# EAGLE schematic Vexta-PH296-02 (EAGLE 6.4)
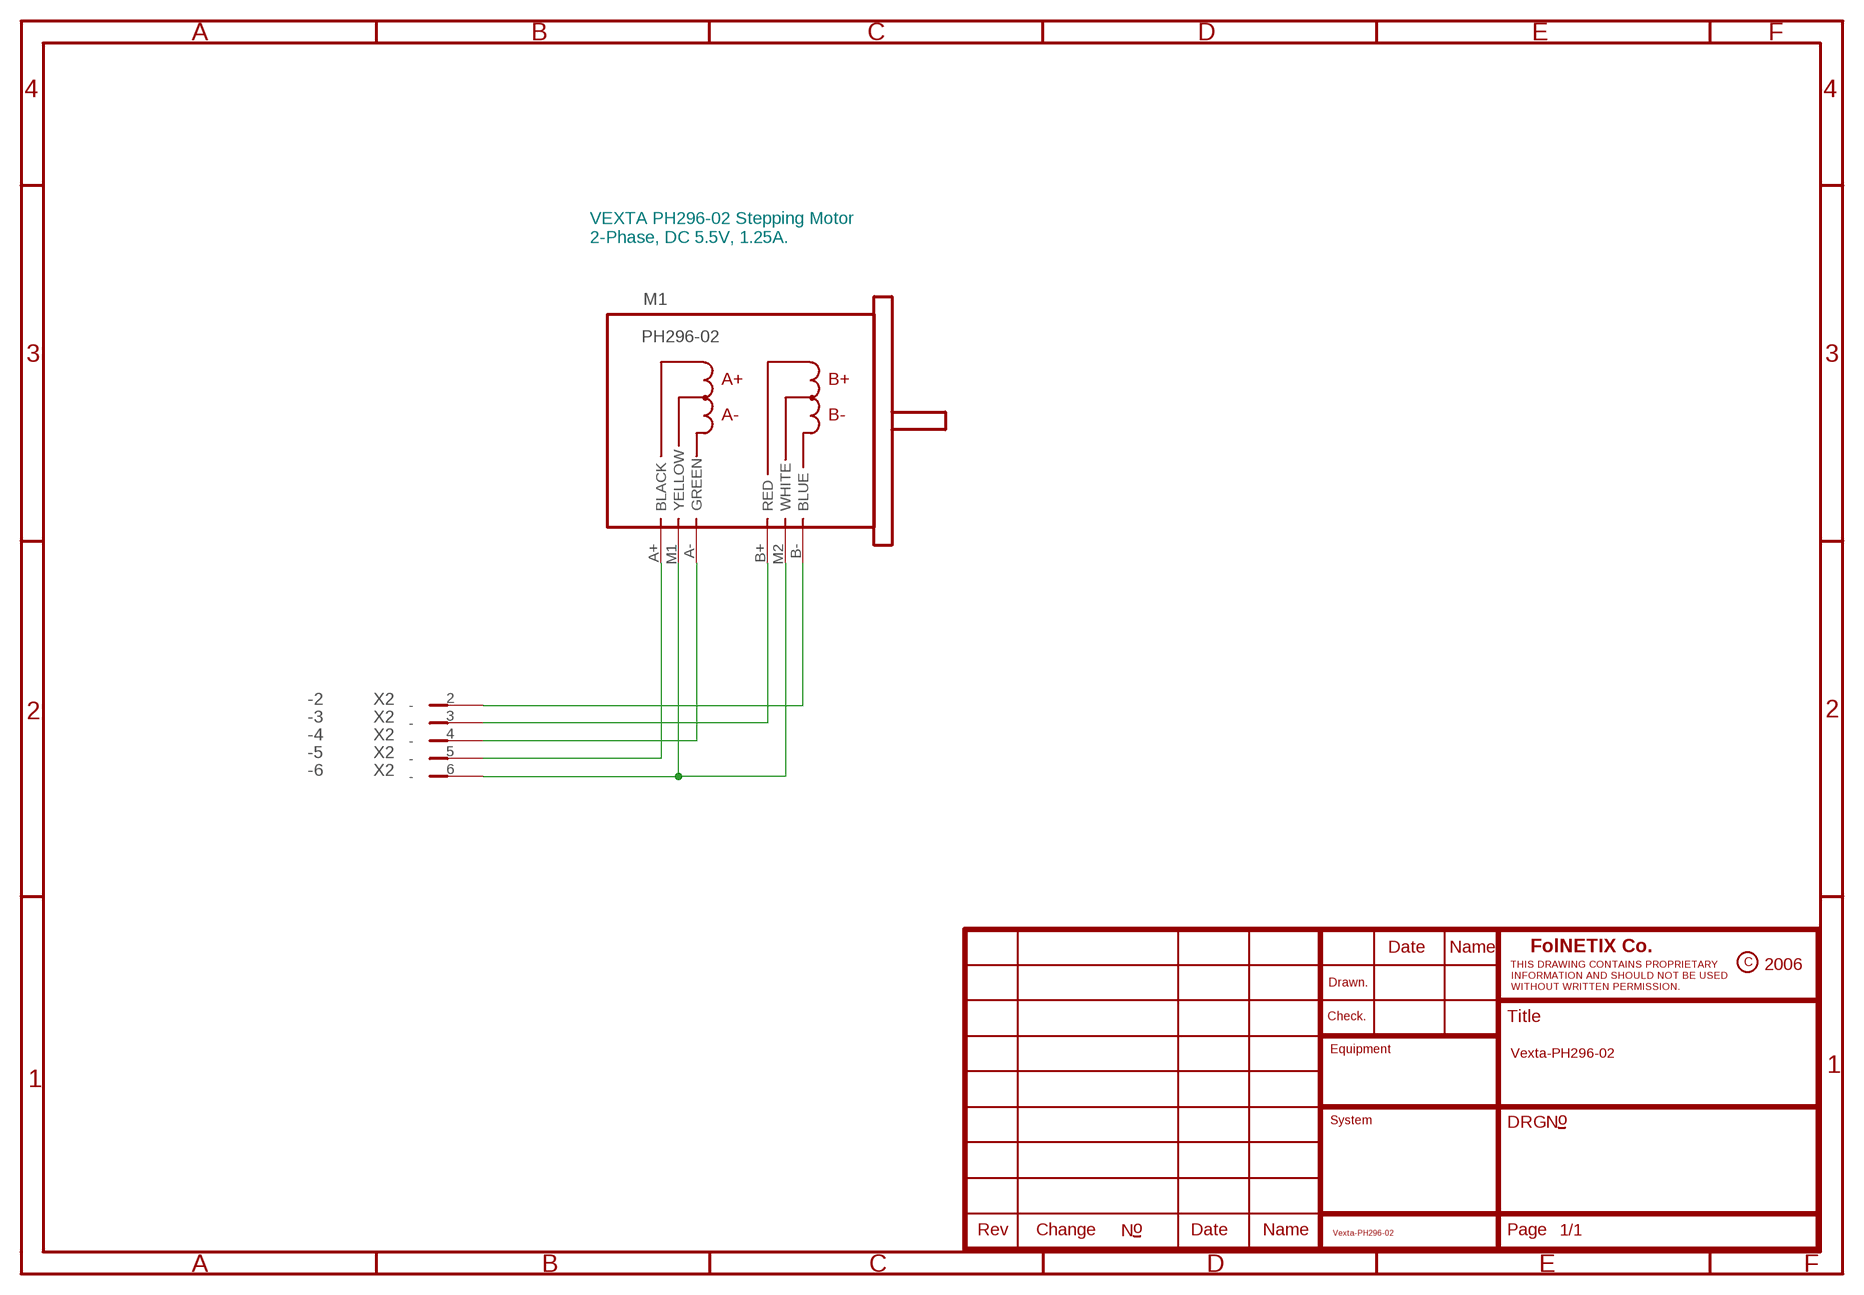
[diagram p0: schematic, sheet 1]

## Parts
M1  PH296-02  [PH296-02]
X2  RIACON-6  [RIACON-6]

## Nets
N$1: M1.B-(BLUE) X2.2
N$2: M1.B+(RED) X2.3
N$3: M1.A-(GREEN) X2.4
N$4: M1.A+(BLACK) X2.5
N$5: M1.M1(YELLOW) M1.M2(WHITE) X2.6
Unconnected: X2.1

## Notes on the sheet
- VEXTA PH296-02 Stepping Motor
  2-Phase, DC 5.5V, 1.25A.

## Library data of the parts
M1 = user1:PH296-02
X2 = con-riacon2:RIACON-6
